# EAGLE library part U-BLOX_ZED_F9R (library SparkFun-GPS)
u-blox ZED-F9K ADR GPS Unit with Real Time Kinematics (RTK) and internal IMU = Automotive Dead Reckoning
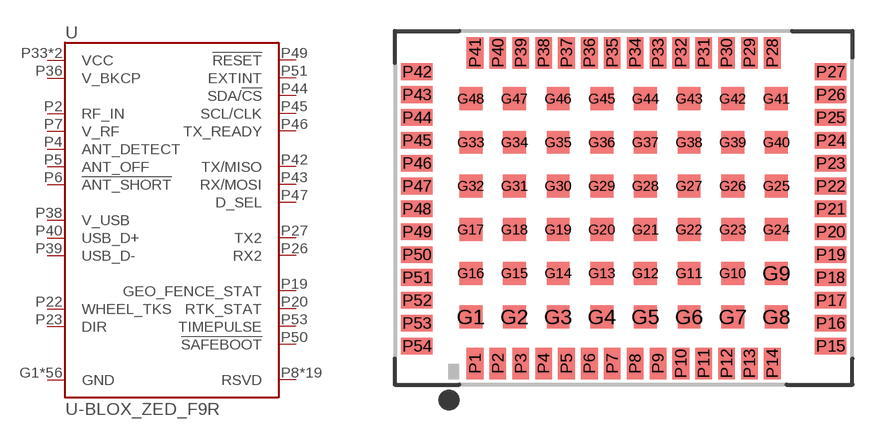
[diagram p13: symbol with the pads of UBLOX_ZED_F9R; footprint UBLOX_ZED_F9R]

Designator prefix U

## U-BLOX_ZED_F9R (PROD_ID: IC-14716)  [UBLOX_ZED_F9R]
G1  GND  pwr
G2  GND  pwr
G3  GND  pwr
G4  GND  pwr
G5  GND  pwr
G6  GND  pwr
G7  GND  pwr
G8  GND  pwr
G9  GND  pwr
G10  GND  pwr
G11  GND  pwr
G12  GND  pwr
G13  GND  pwr
G14  GND  pwr
G15  GND  pwr
G16  GND  pwr
G17  GND  pwr
G18  GND  pwr
G19  GND  pwr
G20  GND  pwr
G21  GND  pwr
G22  GND  pwr
G23  GND  pwr
G24  GND  pwr
G25  GND  pwr
G26  GND  pwr
G27  GND  pwr
G28  GND  pwr
G29  GND  pwr
G30  GND  pwr
G31  GND  pwr
G32  GND  pwr
G33  GND  pwr
G34  GND  pwr
G35  GND  pwr
G36  GND  pwr
G37  GND  pwr
G38  GND  pwr
G39  GND  pwr
G40  GND  pwr
G41  GND  pwr
G42  GND  pwr
G43  GND  pwr
G44  GND  pwr
G45  GND  pwr
G46  GND  pwr
G47  GND  pwr
G48  GND  pwr
P1  GND  pwr
P2  RF_IN  in
P3  GND  pwr
P4  ANT_DETECT  in
P5  ANT_OFF  out
P6  !ANT_SHORT!  out
P7  V_RF  out
P8  RSVD  nc
P9  RSVD  nc
P10  RSVD  nc
P11  RSVD  nc
P12  GND  pwr
P13  RSVD  nc
P14  GND  pwr
P15  RSVD  nc
P16  RSVD  nc
P17  RSVD  nc
P18  RSVD  nc
P19  GEO_FENCE_STAT  out
P20  RTK_STAT  out
P21  RSVD  nc
P22  WHEEL_TKS  in
P23  DIR  in
P24  RSVD  nc
P25  RSVD  nc
P26  RX2  in
P27  TX2  out
P28  RSVD  nc
P29  RSVD  nc
P30  RSVD  nc
P31  RSVD  nc
P32  GND  pwr
P33  VCC  pwr
P34  VCC  pwr
P35  RSVD  nc
P36  V_BKCP  pwr
P37  GND  pwr
P38  V_USB  pwr
P39  USB_D-
P40  USB_D+
P41  GND  pwr
P42  TX/MISO
P43  RX/MOSI
P44  SDA/!CS!
P45  SCL/CLK
P46  TX_READY
P47  D_SEL
P48  GND  pwr
P49  !RESET!
P50  !SAFEBOOT!  in
P51  EXTINT
P52  RSVD  nc
P53  TIMEPULSE  out
P54  RSVD  nc

## Footprint UBLOX_ZED_F9R (pad centres in mm)
u-blox ZED-F9K ADR GPS Unit with Real Time Kinematics (RTK) and internal IMU = Automotive Dead Reckoning Mechanical Specification Physical Module: 22mm x 17mm Peripheral Pad Size: .8mm x 1.5mm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
smd 1.1 x 1.1: G1 -7.312,-5.37; G2 -5.212,-5.37; G3 -3.112,-5.37; G4 -1.012,-5.37; G5 1.088,-5.37; G6 3.188,-5.37; G7 5.288,-5.37; G8 7.388,-5.37; G9 7.388,-3.27; G10 5.288,-3.27; G11 3.188,-3.27; G12 1.088,-3.27; G13 -1.012,-3.27; G14 -3.112,-3.27; G15 -5.212,-3.27; G16 -7.312,-3.27; G17 -7.312,-1.17; G18 -5.212,-1.17; G19 -3.112,-1.17; G20 -1.012,-1.17; G21 1.088,-1.17; G22 3.188,-1.17; G23 5.288,-1.17; G24 7.388,-1.17; G25 7.388,0.93; G26 5.288,0.93; G27 3.188,0.93; G28 1.088,0.93; G29 -1.012,0.93; G30 -3.112,0.93; G31 -5.212,0.93; G32 -7.312,0.93; G33 -7.312,3.03; G34 -5.212,3.03; G35 -3.112,3.03; G36 -1.012,3.03; G37 1.088,3.03; G38 3.188,3.03; G39 5.288,3.03; G40 7.388,3.03; G41 7.388,5.13; G42 5.288,5.13; G43 3.188,5.13; G44 1.088,5.13; G45 -1.012,5.13; G46 -3.112,5.13; G47 -5.212,5.13; G48 -7.312,5.13
smd 0.8 x 1.5: P1 -7.112,-7.62; P2 -6.012,-7.62; P3 -4.912,-7.62; P4 -3.812,-7.62; P5 -2.712,-7.62; P6 -1.612,-7.62; P7 -0.512,-7.62; P8 0.588,-7.62; P9 1.688,-7.62; P10 2.788,-7.62; P11 3.888,-7.62; P12 4.988,-7.62; P13 6.088,-7.62; P14 7.188,-7.62; P28 7.188,7.33; P29 6.088,7.33; P30 4.988,7.33; P31 3.888,7.33; P32 2.788,7.33; P33 1.688,7.33; P34 0.588,7.33; P35 -0.512,7.33; P36 -1.612,7.33; P37 -2.712,7.33; P38 -3.812,7.33; P39 -4.912,7.33; P40 -6.012,7.33; P41 -7.112,7.33
smd 1.5 x 0.8: P15 9.988,-6.77; P16 9.988,-5.67; P17 9.988,-4.57; P18 9.988,-3.47; P19 9.988,-2.37; P20 9.988,-1.27; P21 9.988,-0.17; P22 9.988,0.93; P23 9.988,2.03; P24 9.988,3.13; P25 9.988,4.23; P26 9.988,5.33; P27 9.988,6.43; P42 -9.912,6.43; P43 -9.912,5.33; P44 -9.912,4.23; P45 -9.912,3.13; P46 -9.912,2.03; P47 -9.912,0.93; P48 -9.912,-0.17; P49 -9.912,-1.27; P50 -9.912,-2.37; P51 -9.912,-3.47; P52 -9.912,-4.57; P53 -9.912,-5.67; P54 -9.912,-6.77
